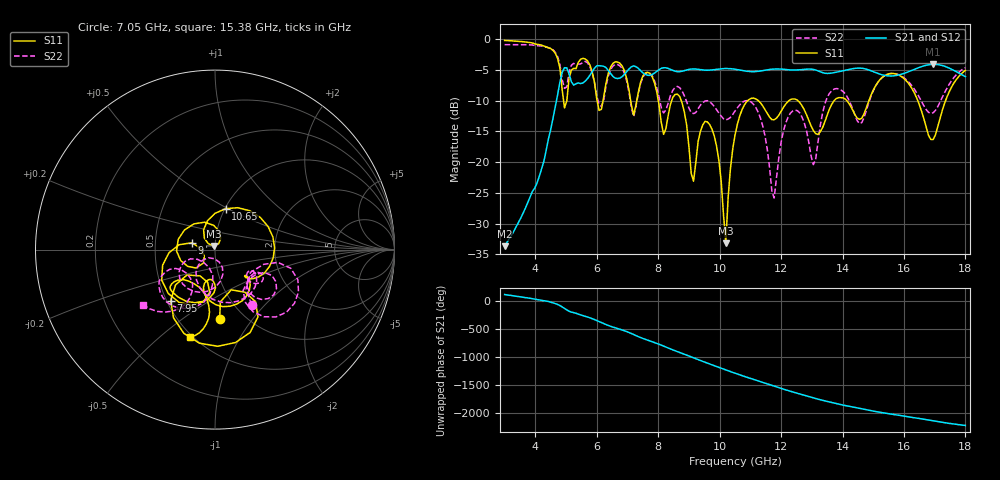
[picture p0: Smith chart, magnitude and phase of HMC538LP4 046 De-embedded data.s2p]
! Chelmsford, MA 01824
! http://www.hittite.com
! Tel: 978-250-3343
! Fax: 978-250-3373
! Device  :  HMC538LP4
! Description:  600 Analog Phase Shifter
! Frequency  :  6.0 GHz - 15.0 GHz
! Package  :  LP4  - 4x4 mm Quad Flatpack No-Lead (QFN) Plastic Package: 24 pin
! Ports  :  2 RF, 1 DC
!  Pin  3  = Rfin  = Port 1
!  Pin  16  = Rfout = Port 2
!  pin  21  = vCTL
! Voltages:  VCTL  = 0 to 5.0 Volts
! Currents :  Vb(V)  Vd(V)  Ib(mA)  Id(mA)
!  0.00  4.60  0.000000	0.484032
! Data:  The device was measured on evaluation board 111296-1.
!  Data was collected using a calibrated network analyzer.
!  The evaluation circuit board was modeled and simulated.This was use
!  to removed the evaluation board circuit from the measured data.
!  The reference plane is the center of the package pin.
! Misc:  Lot #
!Date Measured:  03 - 11 -2009
! Date:  03 - 17 -2009
! Note:
!  Hittite Microwave supplies this data as a sample of measured data at the
!  package pin for this package product.  Your particular data for this product
!  may vary.
!  Data was taken at 25 degrees C.
!  Hittite Microwave reserves the right to change this data at anytime.
# MHz S MA R 50
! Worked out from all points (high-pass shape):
!   201 points, 3 GHz to 18 GHz, reference 50 ohm
!   highest |S21| = -4.08 dB at 16.95 GHz (marker M1); lowest = -33.7 dB at 3 GHz (marker M2)
!   |S21| within 3 dB of the highest: 4.798 GHz to 5.196 GHz (398.8 MHz wide, 7.98 % of centre); 5.559 GHz to end of sweep
!   lowest |S11| = -33.2 dB at 10.2 GHz (marker M3), VSWR 1.04, Z = 49.2 + j1.99 ohm
!   |S11| at or under -10 dB: 8.751 GHz to 10.91 GHz (2.163 GHz wide, 22 % of centre); 11.26 GHz to 12.26 GHz (995.7 MHz wide, 8.47 % of centre); 12.55 GHz to 13.72 GHz (1.174 GHz wide, 8.94 % of centre)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
!   |S22| runs from -25.9 to -0.9 dB; largest |S21 - S12| = 0.0023
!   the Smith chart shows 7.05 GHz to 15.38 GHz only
!   S11 on the Smith chart (normalised r, x): 7.05 GHz: 0.78, -0.70; 7.95 GHz: 0.52, -0.35; 9 GHz: 0.77, +0.06; 10.65 GHz: 1.01, +0.49; 15.38 GHz: 0.49, -0.64
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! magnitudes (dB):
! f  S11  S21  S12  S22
! 3 GHz  -0.2  -33.7  -33.7  -0.9
! 4.875 GHz  -8.3  -5.4  -5.4  -6.6
! 5.55 GHz  -3.1  -7.1  -7.1  -3.8
! 6.075 GHz  -11.6  -4.3  -4.3  -10.6
! 7.05 GHz  -8.3  -4.8  -4.8  -8.7
! 7.95 GHz  -8.5  -5.2  -5.2  -7.8
! 8.025 GHz  -10.6  -5.0  -5.0  -9.3
! 9 GHz  -17.5  -4.9  -4.9  -11.2
! 9.75 GHz  -14.6  -5.0  -5.0  -10.5
! 10.2 GHz  -33.2  -4.8  -4.8  -13.1
! 10.5 GHz  -15.6  -4.9  -4.9  -11.7
! 10.65 GHz  -12.5  -5.0  -5.0  -10.7
! 11.32 GHz  -10.3  -5.2  -5.2  -12.8
! 11.78 GHz  -13.1  -4.8  -4.8  -25.9
! 12.38 GHz  -9.7  -5.0  -5.0  -11.7
! 13.05 GHz  -14.8  -4.9  -4.9  -20.4
! 13.57 GHz  -11.4  -5.5  -5.6  -8.8
! 14.55 GHz  -13.0  -4.7  -4.7  -13.7
! 15.38 GHz  -5.9  -5.9  -5.9  -5.9
! 15.53 GHz  -5.6  -6.0  -6.0  -5.6
! 16.95 GHz  -16.3  -4.1  -4.1  -12.0
! 18 GHz  -5.1  -6.1  -6.1  -4.6
